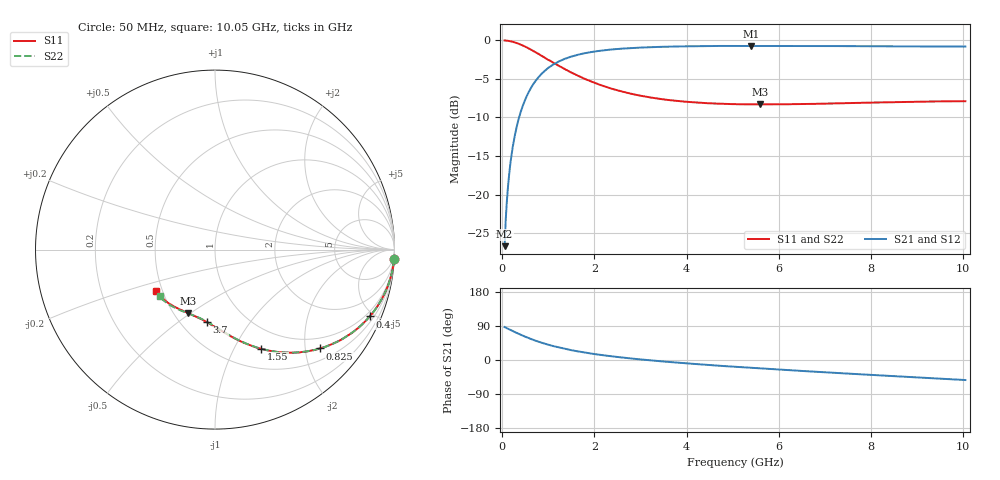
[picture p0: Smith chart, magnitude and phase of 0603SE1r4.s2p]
! AVX Thin Film Operation		Date: August 2001
! Description: Accu-P® Series, Thin Film, SMD, RF Capacitor
! Part Number: 06035J1R4ABT
! 50 MHz  -  10.05 GHz
! Serial Measurements
# mhz S db R 50
!	S11		S21		S12		S22
!	dB	Phase	dB	Phase	dB	Phase	dB	Phase
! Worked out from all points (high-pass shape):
!   401 points, 50 MHz to 10.05 GHz, reference 50 ohm
!   highest |S21| = -0.71 dB at 5.4 GHz (marker M1); lowest = -26.7 dB at 50 MHz (marker M2)
!   |S21| within 3 dB of the highest: 969.8 MHz to end of sweep
!   lowest |S11| = -8.3 dB at 5.6 GHz (marker M3), VSWR 2.25, Z = 29.5 - j24.5 ohm
!   |S11| at or under -10 dB: nowhere
!   |S22| runs from -8.3 to 0.0 dB; largest |S21 - S12| = 0
!   S11 on the Smith chart (normalised r, x): 50 MHz: 1, -38; 400 MHz: 0.75, -4.72; 825 MHz: 0.75, -2.32; 1.55 GHz: 0.73, -1.28; 3.7 GHz: 0.67, -0.65; 10.05 GHz: 0.46, -0.26
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50  -0.01 -3.0  -26.70 87.0  -26.70 87.0  -0.01 -3.0
75  -0.02 -4.6  -23.21 85.4  -23.21 85.4  -0.02 -4.6
125  -0.06 -7.6  -18.89 82.4  -18.89 82.4  -0.06 -7.6
150  -0.08 -9.1  -17.31 80.9  -17.31 80.9  -0.08 -9.1
200  -0.14 -12.1  -14.88 77.9  -14.88 77.9  -0.14 -12.1
300  -0.32 -17.8  -11.54 72.2  -11.54 72.2  -0.32 -17.8
400  -0.55 -23.4  -9.27 66.6  -9.27 66.6  -0.55 -23.4
575  -1.05 -32.3  -6.69 57.7  -6.69 57.7  -1.05 -32.3
825  -1.90 -43.2  -4.51 46.7  -4.51 46.7  -1.90 -43.2
1200  -3.21 -56.1  -2.82 33.8  -2.82 33.8  -3.21 -56.1
1550  -4.32 -65.2  -2.02 24.8  -2.02 24.8  -4.32 -65.1
1725  -4.82 -69.1  -1.74 20.9  -1.74 20.9  -4.82 -69.0
2025  -5.55 -74.8  -1.43 15.3  -1.43 15.3  -5.55 -74.5
2400  -6.31 -80.7  -1.17 9.3  -1.17 9.3  -6.31 -80.4
3400  -7.57 -93.1  -0.85 -2.9  -0.85 -2.9  -7.57 -92.4
3700  -7.80 -96.2  -0.80 -6.0  -0.80 -6.0  -7.79 -95.4
5050  -8.28 -108.6  -0.71 -17.9  -0.71 -17.9  -8.26 -106.6
5400  -8.30 -111.6  -0.71 -20.6  -0.71 -20.6  -8.29 -109.6
5600  -8.31 -112.9  -0.71 -22.2  -0.71 -22.2  -8.29 -110.9
6725  -8.24 -121.4  -0.73 -30.4  -0.73 -30.4  -8.21 -118.4
8400  -8.03 -134.1  -0.77 -41.9  -0.77 -41.9  -8.00 -130.1
10050  -7.89 -144.8  -0.80 -52.9  -0.80 -52.9  -7.86 -139.8
